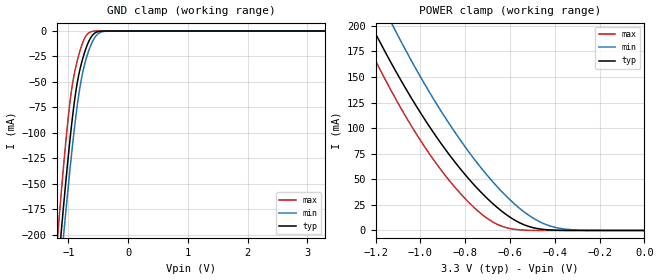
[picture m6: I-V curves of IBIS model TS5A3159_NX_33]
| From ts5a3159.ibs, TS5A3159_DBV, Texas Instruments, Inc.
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[Model]   TS5A3159_NX_33
Model_type  Terminator
| variable   typ   min   max
C_comp   24.31pF   21.95pF   25.22pF
| C_tri-state   24.31pF   21.95pF   25.22pF
[Temperature Range]   40   100   -40
| Ambient temperature   25   85   -40
[Voltage range]   3.3   3   3.6
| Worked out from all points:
|   GND clamp passes 1 mA (typ) near -0.53 V on its own axis
|   POWER clamp passes 1 mA (typ) near -0.45 V on its own axis
[GND Clamp]
| TS5A3159_NX_33
|   Voltage   I(typ)   I(min)   I(max)
-3.3V     -2.159A    -2.094A    -2.278A
-1.185V   -241mA     -268.9mA   -204.5mA
-1.135V   -206.8mA   -235.5mA   -168.7mA
-1.11V    -190.1mA   -219.1mA   -151.4mA
-1.085V   -173.8mA   -203.1mA   -134.6mA
-1V       -121.3mA   -150.8mA   -82.77mA
-925mV    -80.82mA   -108.5mA   -49.34mA
-860mV    -53.34mA   -76.4mA    -30.98mA
-790mV    -33.43mA   -49.18mA   -16.14mA
-635mV    -7.354mA   -15.32mA   -990.2uA
-395mV    -33.34uA   -304uA     -208.9nA
3.3V      972.4pA    423.8uA    72.59pA
[POWER Clamp]
| TS5A3159_NX_33
|   Voltage   I(typ)   I(min)   I(max)
-3.3V     1.641A     1.72A      1.731A
-1.275V   225.1mA    269.1mA    199.8mA
-1.21V    196.6mA    238.6mA    170.3mA
-1.125V   161.6mA    201mA      134.5mA
-1.105V   153.7mA    192.5mA    126.5mA
-960mV    101.7mA    135.3mA    75mA
-800mV    54.51mA    81.68mA    31.11mA
-680mV    26.89mA    48.37mA    8.728mA
-545mV    6.306mA    19.52mA    425.4uA
-455mV    1.141mA    7.226mA    22.25uA
-385mV    209uA      2.361mA    1.543uA
0V        0A         0A         0A
